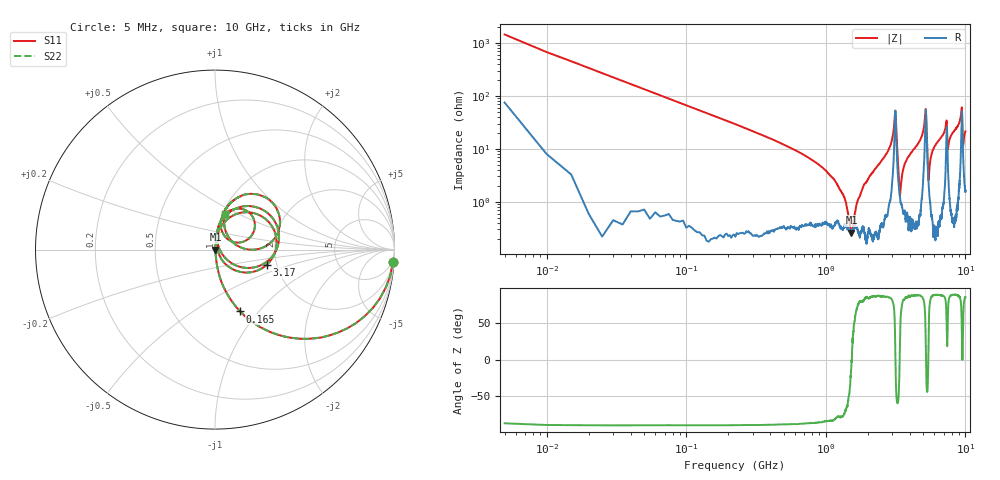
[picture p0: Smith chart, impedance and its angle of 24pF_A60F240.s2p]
! Amotech Co.,Ltd.
! http://www.amotech.co.kr/
! Part Number: A60F240
! These Parameters are Measured in Series Mode Connection
! Operation Temp=25[degC], DC Bias Voltage=0[V]
! Freq. Start=5[MHz] Stop=10[GHz], 2000[Steps]
! Date: Monday, July 20, 2020, 03:38:04
# GHZ S RI R 50.000000
!Freq.(Hz) S11(Real) S11(Imag) S21(Real) S21(Imag) S12(Real) S12(Imag) S22(Real) S22(Imag)
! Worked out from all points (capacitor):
!   2000 points, 5 MHz to 10 GHz, reference 50 ohm
!   read as one part in series: C = 23.8 pF near 55 MHz
!   lowest |Z| = 263 mohm at 1.525 GHz (marker M1)
!   series resonance near 1.536 GHz, so ESL is about 450 pH
!   S11 on the Smith chart (normalised r, x): 5 MHz: 2, -29; 165 MHz: 1.00, -0.80; 3.17 GHz: 1.77, -0.33; 10 GHz: 1.03, +0.43
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0.005  0.9917 -0.0685  0.00832 0.0685  0.00832 0.0685  0.9917 -0.0685
0.07  0.4759 -0.4965  0.5241 0.4965  0.5241 0.4965  0.4759 -0.4965
0.165  0.1401 -0.3446  0.8599 0.3446  0.8599 0.3446  0.1401 -0.3446
1.175  0.00469 -0.0233  0.9953 0.0233  0.9953 0.0233  0.00469 -0.0233
1.525  0.00259 -0.000391  0.9974 0.000391  0.9974 0.000391  0.00259 -0.000391
1.675  0.0033 0.00911  0.9967 -0.00911  0.9967 -0.00911  0.0033 0.00911
3.075  0.1186 0.198  0.8814 -0.198  0.8814 -0.198  0.1186 0.198
3.17  0.2887 -0.085  0.7113 0.085  0.7113 0.085  0.2887 -0.085
3.34  0.0192 -0.0161  0.9808 0.0161  0.9808 0.0161  0.0192 -0.0161
3.405  0.0111 0.00722  0.9889 -0.00722  0.9889 -0.00722  0.0111 0.00722
3.7  0.00835 0.0529  0.9917 -0.0529  0.9917 -0.0529  0.00835 0.0529
5.005  0.0736 0.2018  0.9264 -0.2018  0.9264 -0.2018  0.0736 0.2018
5.215  0.3484 0.0153  0.6516 -0.0153  0.6516 -0.0153  0.3484 0.0153
5.45  0.0216 0.0129  0.9784 -0.0129  0.9784 -0.0129  0.0216 0.0129
5.805  0.0124 0.0889  0.9876 -0.0889  0.9876 -0.0889  0.0124 0.0889
6.67  0.0302 0.1553  0.9698 -0.1553  0.9698 -0.1553  0.0302 0.1553
7.31  0.1852 0.2103  0.8148 -0.2103  0.8148 -0.2103  0.1852 0.2103
7.49  0.0535 0.0756  0.9465 -0.0756  0.9465 -0.0756  0.0535 0.0756
8.335  0.0508 0.21  0.9492 -0.21  0.9492 -0.21  0.0508 0.21
9.38  0.3138 0.2663  0.6862 -0.2663  0.6862 -0.2663  0.3138 0.2663
9.62  0.0806 0.0635  0.9194 -0.0635  0.9194 -0.0635  0.0806 0.0635
10  0.0571 0.1975  0.9429 -0.1975  0.9429 -0.1975  0.0571 0.1975
